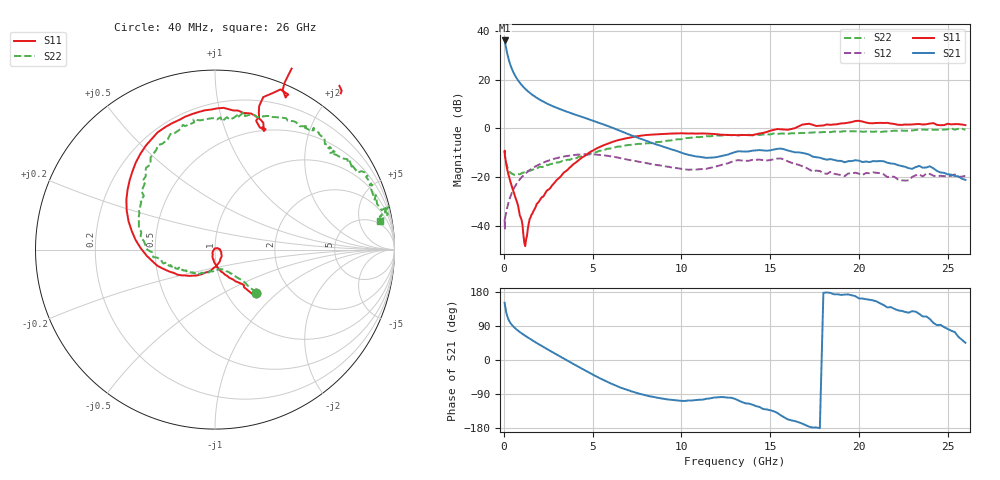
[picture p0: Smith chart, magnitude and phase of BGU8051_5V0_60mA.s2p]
! BGU8051_5V0_60mA
! Date/time Tue Jun 16 11:13:39 2015
! VAR V_out= 5.0010
! VAR I_out= 59.9600
! VAR V_in= 6.3850
! VAR I_in= 0.8226
# MHz S MA R 50
!  Freq-MHz  S11-mag  S11-arg  S21-mag  S21-arg  S12-mag  S12-arg  S22-mag  S22-arg
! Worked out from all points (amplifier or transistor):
!   197 points, 40 MHz to 26 GHz, reference 50 ohm
!   highest |S21| = 36.1 dB at 40 MHz (marker M1)
!   |S21| within 3 dB of that: start of sweep to 120.6 MHz
!   unconditionally stable (mu >= 1): 46.31 MHz to 64.13 MHz; 308.7 MHz to 13.36 GHz; 13.42 GHz to 14.03 GHz
!   at 800 MHz: K = 1.02, MAG = 19.9 dB, |S12| = -21.9 dB
!   at 6.4 GHz: K = 1.30, MAG = 2.4 dB, |S12| = -12.0 dB
!   at 26 GHz: K = -1.47, MSG = -0.8 dB, |S12| = -19.6 dB
!   lowest NFmin = 0.42 dB at 400 MHz
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40  0.3306 -46.6  63.77 151.0  0.01358 31.7  0.3347 -46.9
60  0.2633 -52.4  58.82 145.1  0.008352 49.2  0.2694 -47.8
80  0.2424 -52.1  53.61 139.1  0.01507 37.9  0.2392 -48.1
120  0.1933 -59.1  45.25 128.6  0.01779 44.0  0.1982 -51.7
160  0.1615 -65.2  38.28 120.4  0.02121 51.4  0.1743 -54.1
200  0.1366 -70.8  32.82 114.1  0.02525 54.4  0.1568 -57.4
260  0.1118 -79.3  26.84 106.8  0.03006 58.5  0.1398 -60.7
320  0.09074 -83.9  22.53 101.3  0.03566 61.0  0.1282 -63.8
400  0.07207 -92.2  18.46 95.7  0.04302 62.0  0.1203 -67.4
500  0.05581 -97.5  15.03 90.0  0.05266 62.5  0.1157 -73.7
700  0.03348 -112.6  10.93 81.1  0.07128 61.4  0.1125 -81.7
900  0.0161 -136.1  8.584 73.7  0.08975 58.4  0.1138 -91.2
1200  0.003791 121.6  6.478 63.9  0.1166 53.1  0.1221 -102.3
1550  0.01671 31.6  5.037 53.4  0.1463 46.0  0.1374 -112.9
2700  0.06601 -64.4  2.903 21.7  0.2285 21.0  0.1865 -139.3
4400  0.2516 -146.3  1.714 -23.0  0.2911 -17.4  0.2653 -159.5
6600  0.5902 145.7  0.8686 -73.4  0.2423 -60.1  0.4224 166.5
8800  0.7587 102.7  0.4425 -100.7  0.1729 -78.6  0.5245 141.0
13200  0.7143 67.6  0.3373 -106.6  0.2218 -91.9  0.731 92.0
17400  1.182 50.2  0.2616 -178.2  0.1294 -157.1  0.8187 64.0
21800  1.252 24.4  0.1895 139.6  0.1028 -174.0  0.8746 35.5
26000  1.163 10.6  0.08708 45.6  0.105 169.3  0.9321 9.7
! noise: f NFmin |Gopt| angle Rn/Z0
400  0.4204  0.00611  320.3  0.0514
550  0.4271  0.01711  196  0.0523
950  0.4581  0.06646  188  0.0534
1250  0.4938  0.09782  188.7  0.0536
1600  0.5488  0.129  190.6  0.0538
1900  0.6075  0.1517  192.7  0.0542
2250  0.6894  0.1746  195.5  0.0555
2600  0.7858  0.1946  198.7  0.0584
3300  1.022  0.2302  205.9  0.0708
4000  1.316  0.2671  213.5  0.096
